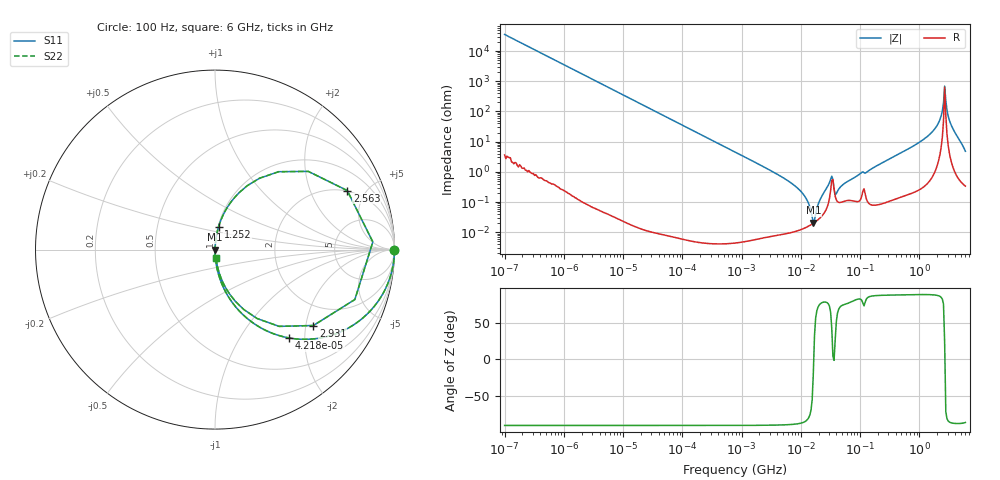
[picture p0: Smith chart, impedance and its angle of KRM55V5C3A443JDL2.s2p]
!Murata Part Number: KRM55V5C3A443JDL2
!These Parameters are Measured in Series Mode Connection
!Data Generated on Jan 08, 2026
!  o--ll--o
!Port1  Port2
!  o------o
!Operation Temp=25[degC], DC Bias Voltage=0[V]
!Freq. Start=100[Hz] Stop=6[GHz] 401[Steps]
# Hz S RI R 50
!Freq.(Hz) S11(Real) S11(Imag) S21(Real) S21(Imag) S12(Real) S12(Imag) S22(Real) S22(Imag)
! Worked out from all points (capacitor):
!   401 points, 100 Hz to 6 GHz, reference 50 ohm
!   read as one part in series: C = 45 nF near 109 Hz
!   lowest |Z| = 20.9 mohm at 16.27 MHz (marker M1)
!   series resonance near 16.52 MHz, so ESL is about 2.1 nH
!   S11 on the Smith chart (normalised r, x): 100 Hz: open; 42.18 kHz: 1.00, -1.68; 1.252 GHz: 1.01, +0.26; 2.563 GHz: 1.97, +3.71; 2.931 GHz: 1.36, -2.21; 6 GHz: 1.01, -0.10
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100  1 -0.00283  8.3e-06 0.00283  8.3e-06 0.00283  1 -0.00283
2008  0.9968 -0.0567  0.00322 0.0567  0.00322 0.0567  0.9968 -0.0567
12041  0.896 -0.3053  0.104 0.3053  0.104 0.3053  0.896 -0.3053
40335  0.4343 -0.4956  0.5657 0.4956  0.5657 0.4956  0.4343 -0.4956
42182  0.4124 -0.4922  0.5876 0.4922  0.5876 0.4922  0.4124 -0.4922
123542  0.0757 -0.2644  0.9243 0.2644  0.9243 0.2644  0.0757 -0.2644
774597  0.00211 -0.0454  0.9979 0.0454  0.9979 0.0454  0.00211 -0.0454
7947587  0.000117 -0.00344  0.9999 0.00344  0.9999 0.00344  0.000117 -0.00344
1.189169e7  0.000142 -0.00146  0.9999 0.00146  0.9999 0.00146  0.000142 -0.00146
1.555665e7  0.000187 -0.000265  0.9998 0.000265  0.9998 0.000265  0.000187 -0.000265
1.626902e7  0.000198 -6.71e-05  0.9998 6.71e-05  0.9998 6.71e-05  0.000198 -6.71e-05
3.184506e7  0.00242 0.00502  0.9976 -0.00502  0.9976 -0.00502  0.00242 0.00502
4.165952e7  0.00103 0.00204  0.999 -0.00204  0.999 -0.00204  0.00103 0.00204
3.124326e8  0.00176 0.0265  0.9982 -0.0265  0.9982 -0.0265  0.00176 0.0265
1.251881e9  0.0197 0.1264  0.9803 -0.1264  0.9803 -0.1264  0.0197 0.1264
2.048624e9  0.1347 0.3176  0.8653 -0.3176  0.8653 -0.3176  0.1347 0.3176
2.34314e9  0.3547 0.434  0.6453 -0.434  0.6453 -0.434  0.3547 0.434
2.562649e9  0.7368 0.329  0.2632 -0.329  0.2632 -0.329  0.7368 0.329
2.931063e9  0.5482 -0.4229  0.4518 0.4229  0.4518 0.4229  0.5482 -0.4229
3.205649e9  0.2353 -0.3843  0.7647 0.3843  0.7647 0.3843  0.2353 -0.3843
3.666503e9  0.0818 -0.2483  0.9182 0.2483  0.9182 0.2483  0.0818 -0.2483
6e9  0.00562 -0.0475  0.9944 0.0475  0.9944 0.0475  0.00562 -0.0475
